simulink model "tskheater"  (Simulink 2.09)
settings: Solver=ode45  StartTime=0.0  StopTime=500  MaxStep=10  RelTol=1e-3  AbsTol=1e-3
undefined symbols (not defined in the file or in its folder): sfunyst
libraries: fuzzy x3

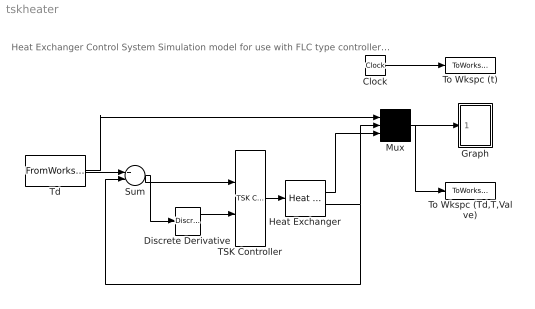
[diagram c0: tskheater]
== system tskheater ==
  note: Heat Exchanger Control System Simulation model for use with FLC type controllers R. Langari 5/18/98
  Clock : Clock
  Discrete Derivative : fuzzy/Discrete Derivative
  Graph : Subsystem  mask(Storage scope.){}
      mask help: Storage scope using MATLAB graph window. Enter plotting ranges and line type.
      mask init:
      | npts = @4; color = @5; ax = [0, @1, @2, @3]; dt=-1;
  Heat Exchanger : fuzzy/Heat Exchanger
  Mux : Mux  Inputs=3
  Sum : Sum  Inputs=+-
  TSK Controller : fuzzy/TSK Controller
  Td : FromWorkspace  VariableName=[t1,Td]
  To Wkspc (Td,T,Valve) : ToWorkspace  VariableName=yout  SampleTime=0
  To Wkspc (t) : ToWorkspace  VariableName=t  SampleTime=0
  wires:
  Heat Exchanger/1 -> Mux/3
  Heat Exchanger/2 -> Mux/2, Sum/2
  Discrete Derivative/1 -> TSK Controller/2
  Sum/1 -> TSK Controller/1, Discrete Derivative/1
  Mux/1 -> Graph/1(x), To Wkspc (Td,T,Valve)/1
  Clock/1 -> To Wkspc (t)/1
  Td/1 -> Mux/1, Sum/1
  TSK Controller/1 -> Heat Exchanger/1

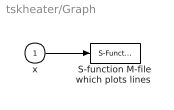
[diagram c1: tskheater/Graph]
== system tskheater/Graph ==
  x : Inport  Port=1  PortWidth=-1  SampleTime=-1
  "S-function M-file which plots lines " : S-Function  LoadFcn=sfunyst([],[],[],'LoadBlock')  FunctionName=sfunyst  Parameters=ax, color, npts, dt
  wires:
  x/1 -> "S-function M-file which plots lines "/1
